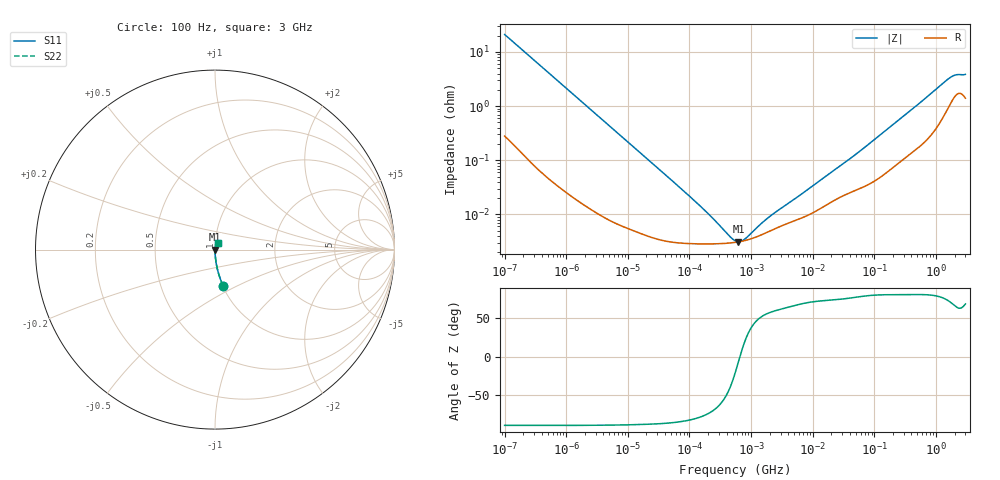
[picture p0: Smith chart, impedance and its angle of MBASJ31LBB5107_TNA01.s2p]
! MBASJ31LBB5107_TNA01  S-PARAMETER MODEL  ( Standard Model )
! Model Generated by TAIYO YUDEN Corporation (http://www.ty-top.com)
! Version 2.0
! TAIYO YUDEN Control No. 231201
! Copyright(c) 2012 TAIYO YUDEN CO.,LTD. All Rights Reserved.
! Product Description (link to TY-COMPAS)
! https://ds.yuden.co.jp/TYCOMPAS/or/detail?pn=MBASJ31LBB5107MTNA01&u=M
! Products Name : Multilayer Ceramic Capacitors
! Characteristics :
!  Capacitance : 100 [uF] , Rated Voltage : 6.3 [V] , TCC : X5R
!  Case Size : 3.2 x 1.6 / 0.126 x 0.063 [mm/inch] , Thickness : 1.6 / 0.063 [mm/inch]
!  (Conditions: Temperature = 25 [degC] , DC Bias Voltage = 0 [V])
! External Node Assignments :
!  1  o---| |---o  2
! GND o---------o GND
! Frequency Range : 100Hz  -  3GHz  [ 401 STEP ]
# MHZ S RI R 50
! Freq[MHz].  S11 Real  S11 Imag  S21 Real  S21 Imag  S12 Real  S12 Imag  S22 Real  S22 Imag
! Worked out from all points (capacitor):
!   401 points, 100 Hz to 3 GHz, reference 50 ohm
!   read as one part in series: C = 75.5 uF near 109 Hz
!   lowest |Z| = 3.13 mohm at 623.2 kHz (marker M1)
!   series resonance near 657.7 kHz, so ESL is about 780 pH
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0.0001  0.0448 -0.2004  0.9552 0.2004  0.9552 0.2004  0.0448 -0.2004
0.000114  0.0353 -0.1782  0.9647 0.1782  0.9647 0.1782  0.0353 -0.1782
0.000175  0.0158 -0.1188  0.9842 0.1188  0.9842 0.1188  0.0158 -0.1188
0.000348  0.00437 -0.0607  0.9956 0.0607  0.9956 0.0607  0.00437 -0.0607
0.000724  0.0012 -0.0294  0.9988 0.0294  0.9988 0.0294  0.0012 -0.0294
0.001788  0.000303 -0.012  0.9997 0.012  0.9997 0.012  0.000303 -0.012
0.031977  3.48e-05 -0.000686  1 0.000686  1 0.000686  3.48e-05 -0.000686
0.203529  2.86e-05 -9.79e-05  1 9.79e-05  1 9.79e-05  2.86e-05 -9.79e-05
0.231582  2.86e-05 -8.33e-05  1 8.33e-05  1 8.33e-05  2.86e-05 -8.33e-05
0.547723  3.05e-05 -1.21e-05  1 1.21e-05  1 1.21e-05  3.05e-05 -1.21e-05
0.623217  3.11e-05 -3.53e-06  1 3.53e-06  1 3.53e-06  3.11e-05 -3.53e-06
1.992254  4.91e-05 7.68e-05  1 -7.68e-05  1 -7.68e-05  4.91e-05 7.68e-05
2.266852  5.25e-05 8.73e-05  0.9999 -8.73e-05  0.9999 -8.73e-05  5.25e-05 8.73e-05
5.135543  7.68e-05 0.000179  0.9999 -0.000179  0.9999 -0.000179  7.68e-05 0.000179
9.794414  0.000106 0.000314  0.9999 -0.000314  0.9999 -0.000314  0.000106 0.000314
48.15176  0.000276 0.00122  0.9997 -0.00122  0.9997 -0.00122  0.000276 0.00122
175.1444  0.000665 0.00399  0.9993 -0.00399  0.9993 -0.00399  0.000665 0.00399
471.3361  0.00166 0.00982  0.9983 -0.00982  0.9983 -0.00982  0.00166 0.00982
1642.185  0.011 0.0306  0.989 -0.0306  0.989 -0.0306  0.011 0.0306
1868.531  0.014 0.0325  0.986 -0.0325  0.986 -0.0325  0.014 0.0325
2126.076  0.0169 0.0332  0.9831 -0.0332  0.9831 -0.0332  0.0169 0.0332
3000  0.0151 0.0349  0.9849 -0.0349  0.9849 -0.0349  0.0151 0.0349
